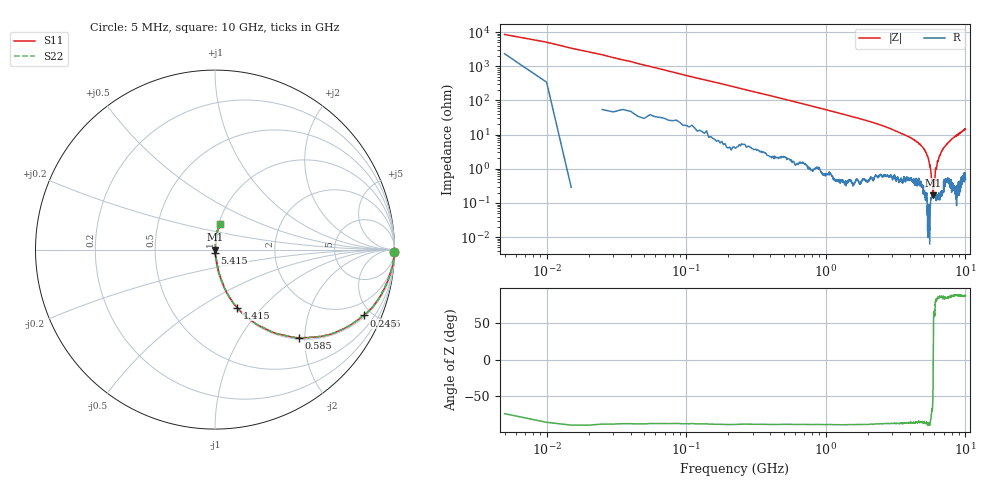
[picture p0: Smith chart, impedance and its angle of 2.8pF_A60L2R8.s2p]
! Amotech Co.,Ltd.
! http://www.amotech.co.kr/
! Part Number: A60L2R8
! These Parameters are Measured in Series Mode Connection
! Operation Temp=25[degC], DC Bias Voltage=0[V]
! Freq. Start=5[MHz] Stop=10[GHz], 2000[Steps]
! Date: Monday, July 14, 2020, 09:30:23
# GHZ S RI R 50.000000
!Freq.(Hz) S11(Real) S11(Imag) S21(Real) S21(Imag) S12(Real) S12(Imag) S22(Real) S22(Imag)
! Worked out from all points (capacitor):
!   2000 points, 5 MHz to 10 GHz, reference 50 ohm
!   read as one part in series: C = 2.95 pF near 55 MHz
!   lowest |Z| = 167 mohm at 5.88 GHz (marker M1)
!   series resonance near 5.879 GHz, so ESL is about 250 pH
!   S11 on the Smith chart (normalised r, x): 5 MHz: open; 245 MHz: 1.09, -4.47; 585 MHz: 1.03, -1.87; 1.415 GHz: 1.01, -0.74; 5.415 GHz: 1.00, -0.04; 10 GHz: 1.01, +0.29
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0.005  0.9967 -0.0112  0.00331 0.0112  0.00331 0.0112  0.9967 -0.0112
0.065  0.9817 -0.1162  0.0183 0.1162  0.0183 0.1162  0.9817 -0.1162
0.095  0.9645 -0.1692  0.0355 0.1692  0.0355 0.1692  0.9645 -0.1692
0.155  0.9204 -0.2599  0.0796 0.2599  0.0796 0.2599  0.9204 -0.2599
0.245  0.8285 -0.3667  0.1715 0.3667  0.1715 0.3667  0.8285 -0.3667
0.585  0.4675 -0.4903  0.5325 0.4903  0.5325 0.4903  0.4675 -0.4903
0.945  0.2475 -0.4251  0.7525 0.4251  0.7525 0.4251  0.2475 -0.4251
1.415  0.1231 -0.3229  0.8769 0.3229  0.8769 0.3229  0.1231 -0.3229
1.675  0.0901 -0.2785  0.9099 0.2785  0.9099 0.2785  0.0901 -0.2785
3.34  0.0174 -0.1132  0.9826 0.1132  0.9826 0.1132  0.0174 -0.1132
5.005  0.00347 -0.0393  0.9965 0.0393  0.9965 0.0393  0.00347 -0.0393
5.415  0.000525 -0.0207  0.9995 0.0207  0.9995 0.0207  0.000525 -0.0207
5.63  0.00113 -0.0103  0.9989 0.0103  0.9989 0.0103  0.00113 -0.0103
5.735  0.00144 -0.00422  0.9986 0.00422  0.9986 0.00422  0.00144 -0.00422
5.88  0.00166 6.26e-05  0.9983 -6.26e-05  0.9983 -6.26e-05  0.00166 6.26e-05
6.015  0.0017 0.00307  0.9983 -0.00307  0.9983 -0.00307  0.0017 0.00307
6.125  0.00165 0.00982  0.9983 -0.00982  0.9983 -0.00982  0.00165 0.00982
6.31  0.00176 0.0165  0.9982 -0.0165  0.9982 -0.0165  0.00176 0.0165
6.67  0.00276 0.0283  0.9972 -0.0283  0.9972 -0.0283  0.00276 0.0283
7.285  0.00693 0.0499  0.9931 -0.0499  0.9931 -0.0499  0.00693 0.0499
8.335  0.00965 0.0839  0.9903 -0.0839  0.9903 -0.0839  0.00965 0.0839
10  0.0257 0.1425  0.9743 -0.1425  0.9743 -0.1425  0.0257 0.1425
